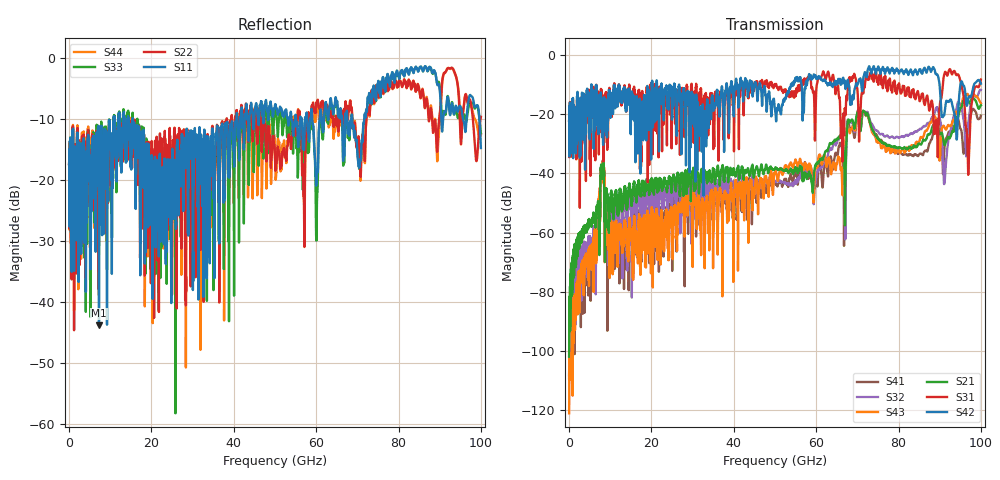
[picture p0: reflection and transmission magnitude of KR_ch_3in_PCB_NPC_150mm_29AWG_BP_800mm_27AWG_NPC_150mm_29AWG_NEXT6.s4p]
# GHz S RI R 45
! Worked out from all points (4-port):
!   4000 points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, 25 MHz to 100 GHz, reference 45 ohm
!   strongest paths, dB at 25 MHz, 25.02 GHz, 50.02 GHz, 75.03 GHz, 100 GHz:
!     S42: -22.2, -20.8, -18.7, -4.1, -9.8
!     S31: -22.2, -16.1, -10.1, -9.6, -8.4
!     S21: -101.8, -43.6, -38.3, -28.3, -17.0
!     S43: -121.0, -58.2, -39.4, -29.6, -16.4
!     S32: -108.0, -52.0, -43.0, -25.8, -11.9
!     S41: -109.2, -66.3, -43.0, -28.0, -20.5
!   lowest |S11| = -43.9 dB at 7.275 GHz (marker M1), VSWR 1.01, Z = 45.2 + j0.542 ohm
!   |S11| at or under -10 dB: start of sweep to 10.89 GHz; 15.45 GHz to 40.64 GHz (25.19 GHz wide, 89.8 % of centre); 68.74 GHz to 71.68 GHz (2.941 GHz wide, 4.19 % of centre)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
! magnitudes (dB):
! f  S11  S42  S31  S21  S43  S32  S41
! 25 MHz  -17.5  -22.2  -22.2  -101.8  -121.0  -108.0  -109.2
! 7.275 GHz  -43.9  -16.4  -25.7  -58.4  -50.6  -51.2  -50.6
! 59.55 GHz  -14.9  -6.9  -16.3  -39.3  -44.4  -47.0  -41.6
! 72.05 GHz  -9.3  -6.9  -7.9  -20.4  -20.6  -20.4  -19.9
! 91.25 GHz  -8.8  -18.6  -6.0  -30.4  -24.8  -42.1  -30.2
! 96.85 GHz  -7.7  -15.2  -36.6  -15.2  -13.4  -24.4  -23.9
! 100 GHz  -14.8  -9.8  -8.4  -17.0  -16.4  -11.9  -20.5
